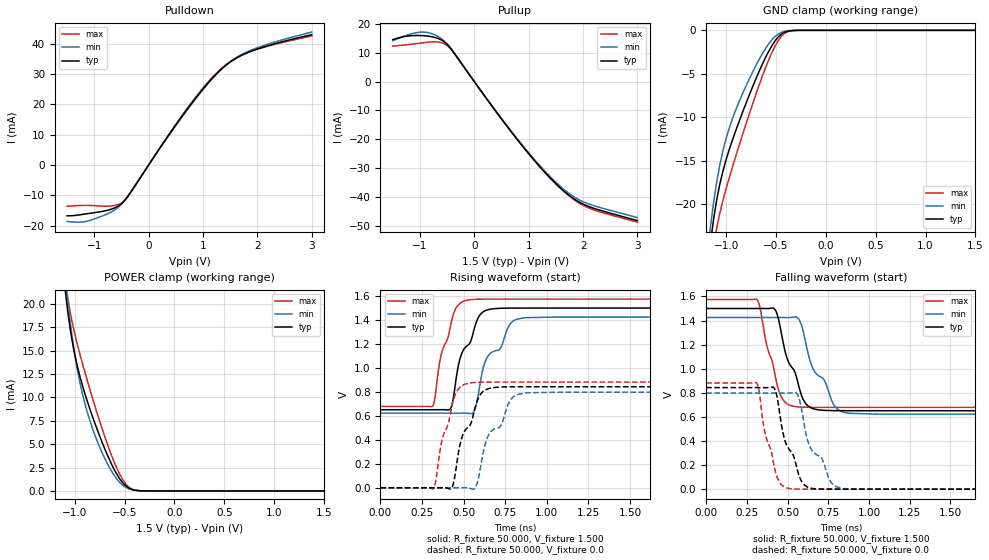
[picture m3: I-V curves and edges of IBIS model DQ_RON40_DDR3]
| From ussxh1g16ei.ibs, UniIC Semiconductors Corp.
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|   Model DQ_RON40_DDR3
[Model] DQ_RON40_DDR3
Model_type I/O
Vinl =  0.615V
Vinh =  0.885V
Vmeas =  0.750V
Rref =  50.000
Vref =  0.750V
C_comp   1.232pF   1.219pF   1.235pF
[Model Spec]
Vinh   0.885V   0.847V   0.922V
Vinl   0.615V   0.577V   0.652V
Vmeas   0.750V   0.712V   0.787V
Vref   0.750V   0.712V   0.787V
Rref   50.000   NA   NA
[Temperature Range]   25.000   95.000   -40.000
[Voltage Range]   1.500V   1.425V   1.575V
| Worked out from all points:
|   slope of the pulldown table from 0 to 0.225 V, typ, clamps not added: 37.1 ohm
|   slope of the pullup table from 0 to 0.225 V, typ, clamps not added: 38 ohm
|   GND clamp passes 1 mA (typ) near -0.49 V on its own axis
|   POWER clamp passes 1 mA (typ) near -0.53 V on its own axis
|   rising waveform, R_fixture 50.000, V_fixture 1.500: 20-80 % time 119ps typ, 159ps min, 90.7ps max; typ from 0.651 V to 1.5 V
|   rising waveform, R_fixture 50.000, V_fixture 0.0: 20-80 % time 115ps typ, 152ps min, 88.6ps max; typ from 0 V to 0.843 V
|   falling waveform, R_fixture 50.000, V_fixture 1.500: 20-80 % time 119ps typ, 155ps min, 92ps max; typ from 1.5 V to 0.651 V
|   falling waveform, R_fixture 50.000, V_fixture 0.0: 20-80 % time 112ps typ, 147ps min, 84.6ps max; typ from 0.843 V to 0 V
[Pulldown]
|Voltage   I(typ)   I(min)   I(max)
-1.5V     -16.71mA   -18.54mA   -13.56mA
-1.086V   -15.9mA    -18.26mA   -13.28mA
-718mV    -14.7mA    -15.72mA   -13.5mA
-488mV    -12.55mA   -12.66mA   -12.36mA
-350mV    -9.492mA   -9.352mA   -9.618mA
340mV     9.085mA    8.939mA    9.236mA
754mV     19.45mA    19.22mA    19.73mA
1.076V    26.66mA    26.47mA    26.97mA
1.352V    31.79mA    31.75mA    32.03mA
1.582V    34.87mA    35.02mA    35mA
1.904V    37.6mA     37.96mA    37.58mA
3V        42.92mA    43.77mA    42.48mA
[Pullup]
|Voltage   I(typ)   I(min)   I(max)
-1.5V     14.53mA    14.14mA    12.29mA
-1.14V    15.91mA    16.63mA    12.98mA
-910mV    15.87mA    17.12mA    13.51mA
-680mV    15.02mA    15.77mA    13.74mA
-496mV    12.85mA    12.92mA    12.45mA
-358mV    9.588mA    9.523mA    9.456mA
746mV     -19.04mA   -18.81mA   -18.92mA
1.16V     -28.56mA   -28.18mA   -28.48mA
1.528V    -35.91mA   -35.37mA   -35.95mA
1.804V    -40.27mA   -39.58mA   -40.5mA
2.034V    -42.74mA   -41.89mA   -43.19mA
3V        -48.17mA   -47.14mA   -48.71mA
[GND_clamp]
|Voltage   I(typ)   I(min)   I(max)
-1.5V     -77.15mA   -73.99mA   -84.26mA
-1.159V   -24.58mA   -22.75mA   -27.74mA
-1.128V   -21.88mA   -19.96mA   -25.03mA
-1.097V   -19.64mA   -17.59mA   -22.88mA
-1.066V   -17.82mA   -15.61mA   -21.14mA
-1.004V   -15mA      -12.58mA   -18.36mA
-880mV    -10.79mA   -8.48mA    -13.61mA
-632mV    -3.776mA   -2.594mA   -5.119mA
-477mV    -756.2uA   -431.9uA   -1.164mA
-415mV    -225.6uA   -131.2uA   -354.1uA
-322mV    -19.15uA   -14.82uA   -24.1uA
1.5V      0A         0A         0A
[POWER_clamp]
|Voltage   I(typ)   I(min)   I(max)
-1.5V     91.1mA     92.64mA    94.46mA
-1.104V   22.28mA    23.97mA    23.43mA
-1.073V   19.41mA    20.63mA    20.89mA
-1.042V   17.07mA    17.76mA    18.91mA
-980mV    13.62mA    13.3mA     15.93mA
-918mV    11.11mA    10.16mA    13.45mA
-856mV    9.013mA    7.787mA    11.15mA
-670mV    3.78mA     2.864mA    4.931mA
-577mV    1.775mA    1.269mA    2.414mA
-484mV    502.3uA    362.1uA    693.5uA
-329mV    12.96uA    15.92uA    9.805uA
1.5V      0A         0A         0A
[Ramp]
| variable   typ   min   max
dV/dt_r   0.506/0.115n   0.479/0.152n   0.529/88.650p
dV/dt_f   0.509/0.119n   0.481/0.155n   0.537/91.863p
R_load = 50.000
[Rising Waveform]
R_fixture= 50.000
V_fixture= 1.500
V_fixture_min= 1.425
V_fixture_max= 1.575
|time   V(typ)   V(min)   V(max)
0s        651.3mV    622.6mV    679.2mV
316ps     651.4mV    622.6mV    686.2mV
359ps     651.6mV    622.6mV    1.074V
421ps     661.1mV    622.6mV    1.352V
478ps     1.079V     622.8mV    1.54V
513ps     1.177V     622.7mV    1.563V
563ps     1.324V     641mV      1.572V
612ps     1.463V     970mV      1.574V
815ps     1.5V       1.405V     1.575V
3ns       1.5V       1.425V     1.575V
[Rising Waveform]
R_fixture= 50.000
V_fixture= 0.0
V_fixture_min= 0.0
V_fixture_max= 0.0
|time   V(typ)   V(min)   V(max)
0s        141.7nV    576.3nV    59.6nV
321ps     -20.62uV   11.11uV    -1.073mV
366ps     524.3uV    23.65uV    375.3mV
428ps     -2.137mV   -14.31uV   675.9mV
490ps     423.8mV    588.9uV    851.9mV
531ps     509.9mV    -1.88mV    873mV
573ps     691mV      7.823mV    879.3mV
615ps     801.6mV    278.2mV    881.2mV
828ps     843.1mV    780.4mV    882mV
3ns       843.3mV    797.6mV    882mV
[Falling Waveform]
R_fixture= 50.000
V_fixture= 1.500
V_fixture_min= 1.425
V_fixture_max= 1.575
|time   V(typ)   V(min)   V(max)
0s        1.5V       1.425V     1.575V
315ps     1.5V       1.425V     1.569V
423ps     1.49V      1.425V     946.4mV
469ps     1.243V     1.425V     747.1mV
534ps     998.6mV    1.428V     689.2mV
583ps     788.2mV    1.371V     681.6mV
626ps     690.5mV    1.126V     679.9mV
782ps     652.1mV    704.5mV    679.2mV
847ps     651.5mV    637.3mV    679.2mV
3ns       651.3mV    622.6mV    679.2mV
[Falling Waveform]
R_fixture= 50.000
V_fixture= 0.0
V_fixture_min= 0.0
V_fixture_max= 0.0
|time   V(typ)   V(min)   V(max)
0s        843.3mV    797.6mV    882mV
311ps     843.3mV    797.6mV    880.7mV
359ps     842.8mV    797.6mV    480.6mV
419ps     836.5mV    797.6mV    181.5mV
499ps     352.1mV    797.2mV    8.932mV
562ps     149.8mV    783.7mV    768.1uV
609ps     28.59mV    485.6mV    121.8uV
762ps     102.3uV    68.3mV     485.9nV
841ps     5.732uV    4.82mV     196.4nV
3ns       233nV      662.5nV    129.3nV
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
